(* Logix 5000 AddOnInstructionDefinition export AMCI_3204_AOP_Immediate_Stop; software revision 20.03 *)

ADD_ON_INSTRUCTION AMCI_3204_AOP_Immediate_Stop   (* revision 1.0, vendor AMCI, ExecuteEnableInFalse *)
VAR_INPUT
   channel_number : INT; {required}
END_VAR
VAR_IN_OUT
   AMCI_3204_output_data : AM:1756_3204:O:0; {required}
END_VAR
VAR
   command_data_block : DINT[8]; {access None}
END_VAR

ROUTINE EnableInFalse   (* ladder *)
END_ROUTINE

ROUTINE Logic   (* ladder *)
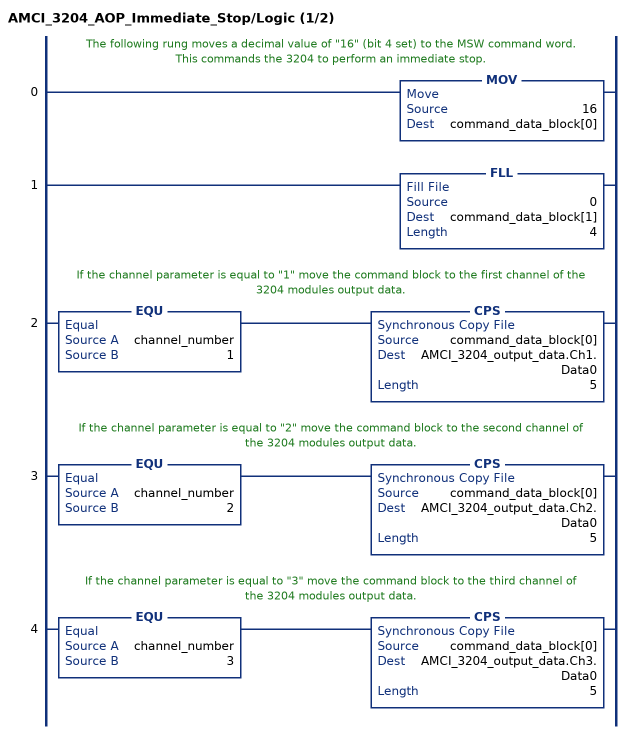
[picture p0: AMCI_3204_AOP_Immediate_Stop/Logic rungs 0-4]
   // The following rung moves a decimal value of "16" (bit 4 set) to the MSW command word.  This commands the 3204 to perform an immediate stop.
   0: MOV(16,command_data_block[0]);
   1: FLL(0,command_data_block[1],4);
   // If the channel parameter is equal to "1" move the command block to the first channel of the 3204 modules output data.
   2: EQU(channel_number,1)CPS(command_data_block[0],AMCI_3204_output_data.Ch1.Data0,5);
   // If the channel parameter is equal to "2" move the command block to the second channel of the 3204 modules output data.
   3: EQU(channel_number,2)CPS(command_data_block[0],AMCI_3204_output_data.Ch2.Data0,5);
   // If the channel parameter is equal to "3" move the command block to the third channel of the 3204 modules output data.
   4: EQU(channel_number,3)CPS(command_data_block[0],AMCI_3204_output_data.Ch3.Data0,5);
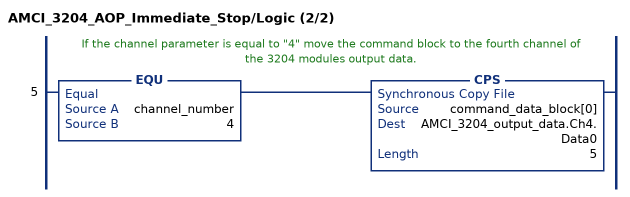
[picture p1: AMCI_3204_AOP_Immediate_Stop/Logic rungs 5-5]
   // If the channel parameter is equal to "4" move the command block to the fourth channel of the 3204 modules output data.
   5: EQU(channel_number,4)CPS(command_data_block[0],AMCI_3204_output_data.Ch4.Data0,5);
END_ROUTINE
END_ADD_ON_INSTRUCTION
